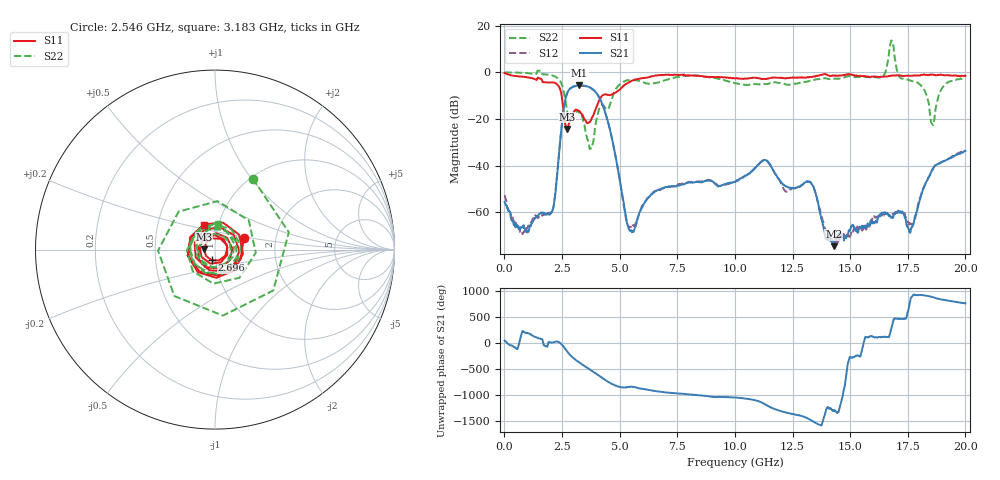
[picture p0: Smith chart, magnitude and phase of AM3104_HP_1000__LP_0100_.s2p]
!Created with skrf (http://scikit-rf.org).
# Hz S RI R 50.0
!freq ReS11 ImS11 ReS21 ImS21 ReS12 ImS12 ReS22 ImS22
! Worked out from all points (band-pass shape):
!   1601 points, 10 MHz to 20 GHz, reference 50 ohm
!   highest |S21| = -5.64 dB at 3.246 GHz (marker M1); lowest = -74.5 dB at 14.29 GHz (marker M2)
!   |S21| within 3 dB of the highest: 2.738 GHz to 3.975 GHz (1.238 GHz wide, 36.9 % of centre)
!   lowest |S11| = -24.3 dB at 2.721 GHz (marker M3), VSWR 1.13, Z = 44.2 + j0.117 ohm
!   |S11| at or under -10 dB: 2.484 GHz to 4.246 GHz (1.762 GHz wide, 52.4 % of centre)
!   |S22| runs from -33.0 to 13.6 dB; largest |S21 - S12| = 0.028
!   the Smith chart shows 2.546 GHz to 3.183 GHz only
!   S11 on the Smith chart (normalised r, x): 2.546 GHz: 1.37, +0.19; 2.696 GHz: 0.96, -0.12; 3.183 GHz: 0.86, +0.24
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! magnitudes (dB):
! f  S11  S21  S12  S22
! 10 MHz  -0.4  -55.6  -52.6  0.0
! 772.1 MHz  -1.9  -66.5  -69.0  -0.2
! 2.034 GHz  -4.3  -60.2  -60.1  -1.2
! 2.546 GHz  -15.2  -17.8  -17.9  -7.0
! 2.696 GHz  -24.1  -9.7  -9.7  -15.2
! 2.721 GHz  -24.3  -9.0  -9.0  -16.9
! 3.183 GHz  -16.4  -5.7  -5.8  -16.8
! 3.246 GHz  -16.8  -5.6  -5.7  -17.3
! 3.346 GHz  -17.7  -5.7  -5.8  -18.1
! 3.758 GHz  -20.5  -6.7  -6.8  -32.5
! 4.358 GHz  -9.4  -16.7  -16.7  -15.0
! 5.445 GHz  -4.1  -68.0  -66.4  -3.4
! 6.682 GHz  -1.2  -50.4  -50.6  -4.4
! 10.01 GHz  -2.7  -47.1  -47.0  -4.7
! 11.3 GHz  -2.9  -37.6  -37.8  -5.1
! 13.34 GHz  -2.1  -48.0  -48.0  -3.5
! 14.29 GHz  -1.4  -74.5  -73.0  -2.7
! 16.68 GHz  -1.6  -61.5  -61.4  7.2
! 17.64 GHz  -1.4  -67.1  -65.3  -3.7
! 18.56 GHz  -0.9  -41.7  -42.0  -22.2
! 19.03 GHz  -1.2  -38.2  -38.2  -6.3
! 20 GHz  -1.5  -33.8  -33.3  -2.5
